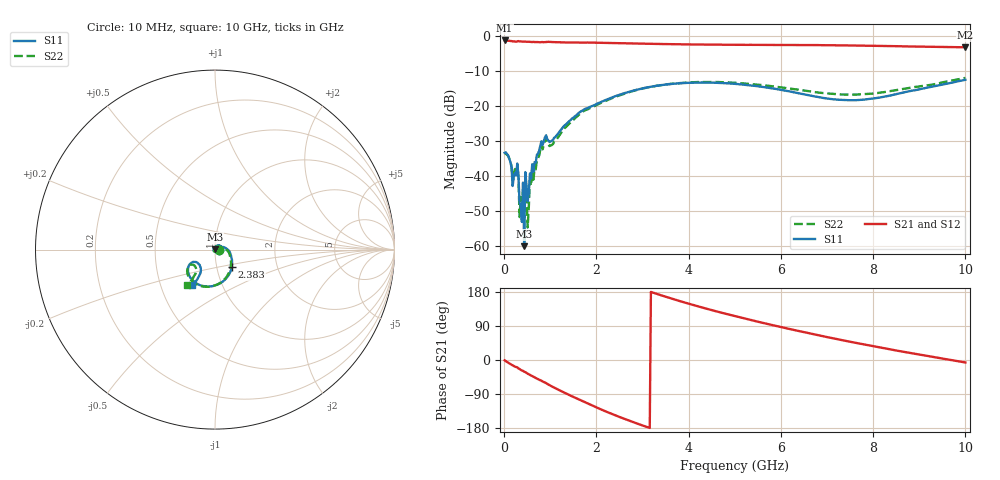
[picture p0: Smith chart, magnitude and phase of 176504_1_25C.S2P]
!  2-Port S-parameters saved by WinCal
! VAR MeasName=S-Parameters (CALIBRATED_DATA) read from VNA (N5242A)
! VAR MeasDate=2017-11-2 16:03:05
! VAR NAME=176504_1_25C
! VAR FILENAME=176504_1_25C.S2P
! VAR DATE=2017-11-2 16:03:05
! VAR PHYS_PORTS=2,3
# Hz S DB R 50
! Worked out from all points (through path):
!   401 points, 10 MHz to 10 GHz, reference 50 ohm
!   highest |S21| = -1.34 dB at 10 MHz (marker M1); lowest = -3.3 dB at 10 GHz (marker M2)
!   lowest |S11| = -60.0 dB at 434.6 MHz (marker M3), VSWR 1.00, Z = 49.9 + j0.0587 ohm
!   |S11| at or under -10 dB: start of sweep to end of sweep
!   |S22| runs from -54.7 to -12.0 dB; largest |S21 - S12| = 0.0057
!   S11 on the Smith chart (normalised r, x): 10 MHz: 1.04, -0.00; 2.383 GHz: 1.18, -0.24; 10 GHz: 0.72, -0.30
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1e7  -33.42 -2.6  -1.34 -0.9  -1.35 -0.9  -33.62 -3.2
8.4925e7  -34.08 -38.6  -1.41 -6.9  -1.41 -6.9  -34.26 -41.3
2.098e8  -40.11 -95.1  -1.58 -15.8  -1.58 -15.8  -39.25 -99.8
2.5975e8  -39.88 146.0  -1.72 -18.5  -1.72 -18.5  -39.68 154.0
3.5965e8  -48.08 -66.2  -1.61 -26.0  -1.61 -26.0  -45.97 -84.8
3.84625e8  -53.11 -172.8  -1.66 -27.6  -1.66 -27.6  -48.80 -153.3
4.34575e8  -60.03 143.9  -1.67 -31.1  -1.67 -31.1  -53.37 -142.6
4.84525e8  -42.73 89.8  -1.71 -34.1  -1.71 -34.1  -45.12 101.2
5.095e8  -47.26 59.7  -1.68 -36.0  -1.68 -36.0  -54.70 61.9
5.34475e8  -44.96 85.0  -1.72 -37.7  -1.72 -37.7  -48.96 103.8
6.094e8  -36.65 83.3  -1.80 -42.4  -1.79 -42.4  -37.91 88.9
8.5915e8  -30.08 47.3  -1.84 -58.1  -1.84 -58.1  -31.14 46.2
1.033975e9  -29.98 22.8  -1.79 -69.7  -1.79 -69.7  -31.18 18.2
1.683325e9  -21.46 -10.3  -1.95 -107.7  -1.95 -107.7  -21.88 -13.4
2.382625e9  -17.37 -46.4  -2.08 -144.6  -2.08 -144.6  -17.55 -48.8
3.35665e9  -14.19 -85.9  -2.34 172.6  -2.35 172.6  -14.17 -87.0
4.180825e9  -13.35 -112.7  -2.49 142.3  -2.51 142.4  -13.22 -112.5
5.005e9  -13.72 -133.1  -2.57 115.7  -2.57 115.8  -13.41 -131.9
6.678325e9  -17.17 -150.4  -2.65 68.9  -2.67 69.0  -15.96 -148.2
7.55245e9  -18.38 -137.6  -2.79 46.9  -2.79 47.0  -16.80 -140.2
8.35165e9  -17.10 -124.2  -2.94 28.4  -2.97 28.6  -15.84 -130.5
1e10  -12.56 -122.7  -3.29 -6.5  -3.31 -6.3  -12.03 -129.0
